(* Logix 5000 AddOnInstructionDefinition export Banner_K50ProTouch_Param_v4; software revision 33.00; part 2 of 2 *)
(* tags used below, declared in another part *)
   K50ProTouch : Banner_K50ProTouch_v4;
   Port_Data : Banner_IOL_Port_v4;
   Port : DINT;
   Local_Control : DINT;
   Command_Being_Processed : BOOL;
   Update_Archive : BOOL;
   Index_Write_Inprocess : INT;
   Inprocess_Index : DINT;
   SP_Index : DINT;   // State Parameters Index
   SP_W_Index : DINT;
(* Banner_K50ProTouch_Param_v4, continued *)

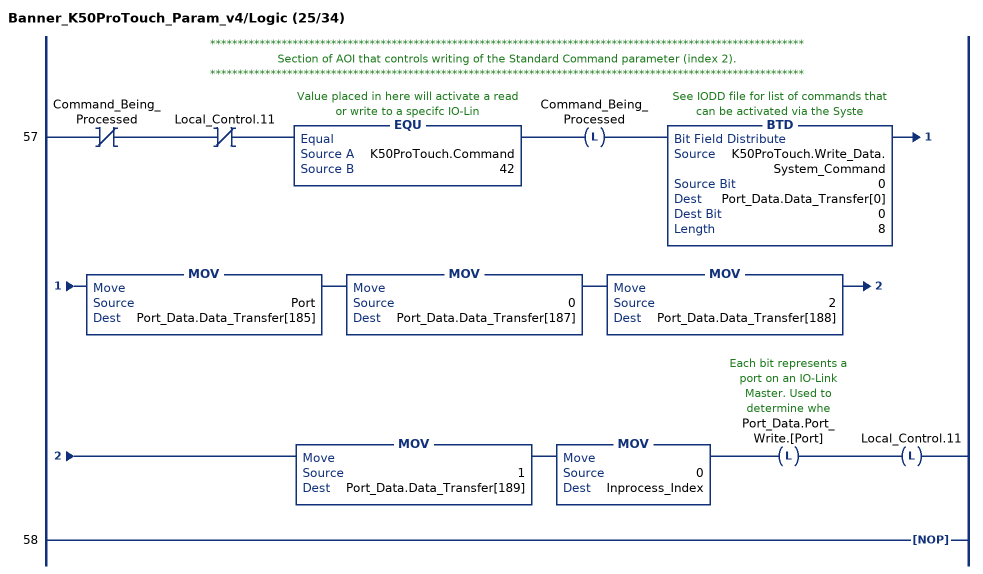
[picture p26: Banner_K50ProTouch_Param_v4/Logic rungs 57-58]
   // ************************************************************************************************************
   // Section of AOI that controls writing of the Standard Command parameter (index 2).
   // ************************************************************************************************************
   57: XIO(Command_Being_Processed)XIO(Local_Control.11)EQU(K50ProTouch.Command,42)OTL(Command_Being_Processed)BTD(K50ProTouch.Write_Data.System_Command,0,Port_Data.Data_Transfer[0],0,8)MOV(Port,Port_Data.Data_Transfer[185])MOV(0,Port_Data.Data_Transfer[187])MOV(2,Port_Data.Data_Transfer[188])MOV(1,Port_Data.Data_Transfer[189])MOV(0,Inprocess_Index)OTL(Port_Data.Port_Write.[Port])OTL(Local_Control.11);
   58: NOP();
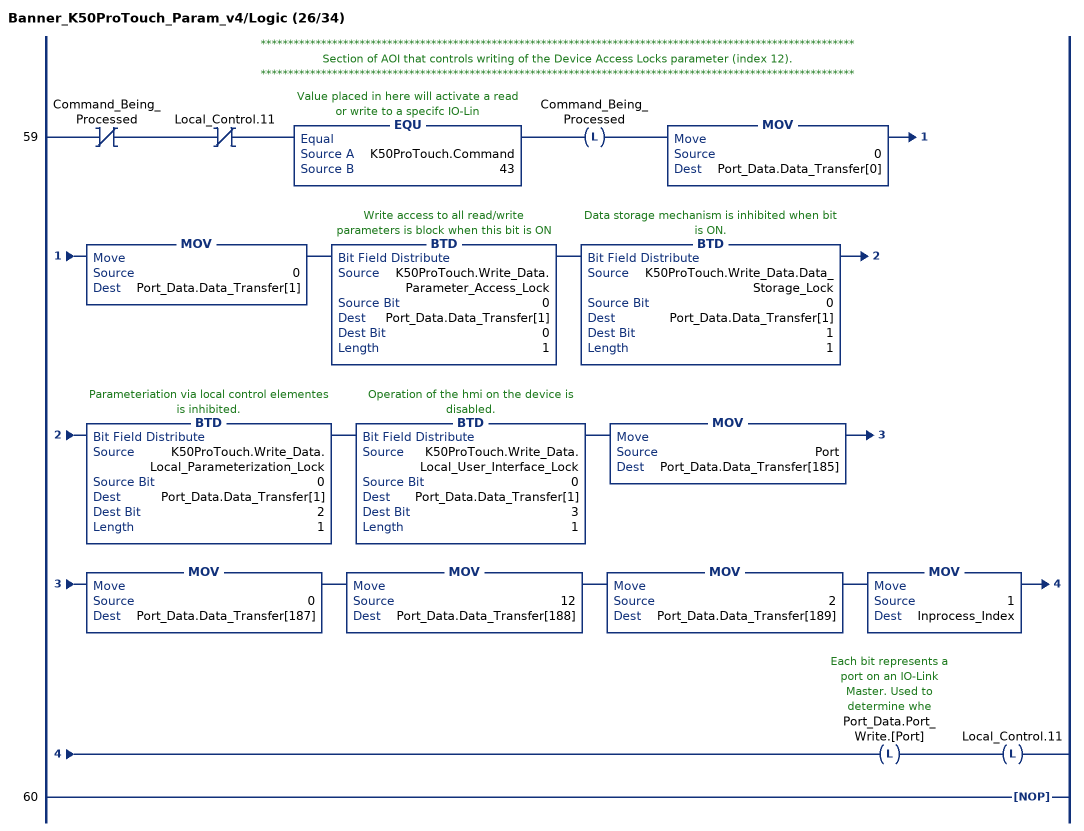
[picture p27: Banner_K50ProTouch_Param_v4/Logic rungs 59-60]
   // ************************************************************************************************************
   // Section of AOI that controls writing of the Device Access Locks parameter (index 12).
   // ************************************************************************************************************
   59: XIO(Command_Being_Processed)XIO(Local_Control.11)EQU(K50ProTouch.Command,43)OTL(Command_Being_Processed)MOV(0,Port_Data.Data_Transfer[0])MOV(0,Port_Data.Data_Transfer[1])BTD(K50ProTouch.Write_Data.Parameter_Access_Lock,0,Port_Data.Data_Transfer[1],0,1)BTD(K50ProTouch.Write_Data.Data_Storage_Lock,0,Port_Data.Data_Transfer[1],1,1)BTD(K50ProTouch.Write_Data.Local_Parameterization_Lock,0,Port_Data.Data_Transfer[1],2,1)BTD(K50ProTouch.Write_Data.Local_User_Interface_Lock,0,Port_Data.Data_Transfer[1],3,1)MOV(Port,Port_Data.Data_Transfer[185])MOV(0,Port_Data.Data_Transfer[187])MOV(12,Port_Data.Data_Transfer[188])MOV(2,Port_Data.Data_Transfer[189])MOV(1,Inprocess_Index)OTL(Port_Data.Port_Write.[Port])OTL(Local_Control.11);
   60: NOP();
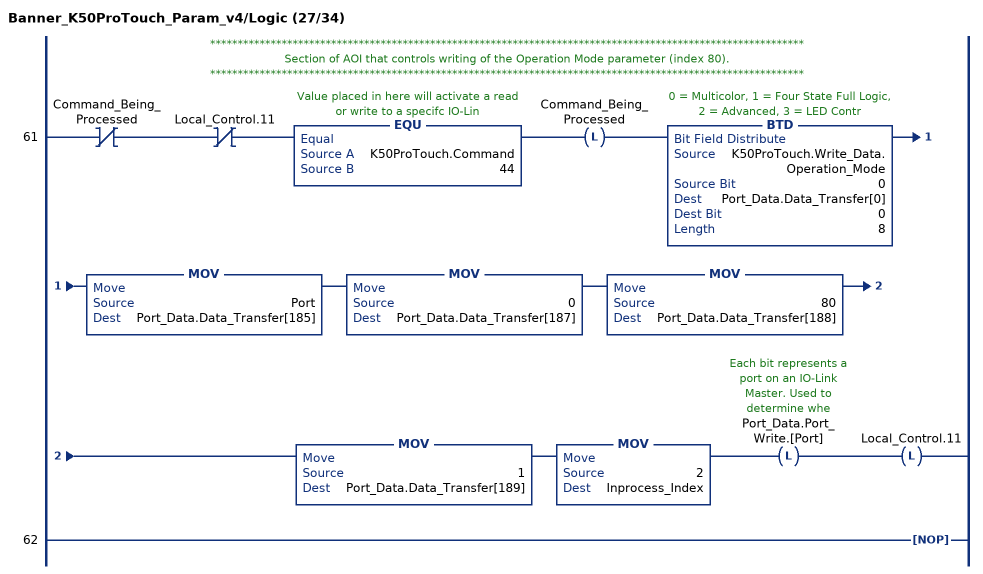
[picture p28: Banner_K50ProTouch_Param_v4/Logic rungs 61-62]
   // ************************************************************************************************************
   // Section of AOI that controls writing of the Operation Mode parameter (index 80).
   // ************************************************************************************************************
   61: XIO(Command_Being_Processed)XIO(Local_Control.11)EQU(K50ProTouch.Command,44)OTL(Command_Being_Processed)BTD(K50ProTouch.Write_Data.Operation_Mode,0,Port_Data.Data_Transfer[0],0,8)MOV(Port,Port_Data.Data_Transfer[185])MOV(0,Port_Data.Data_Transfer[187])MOV(80,Port_Data.Data_Transfer[188])MOV(1,Port_Data.Data_Transfer[189])MOV(2,Inprocess_Index)OTL(Port_Data.Port_Write.[Port])OTL(Local_Control.11);
   62: NOP();
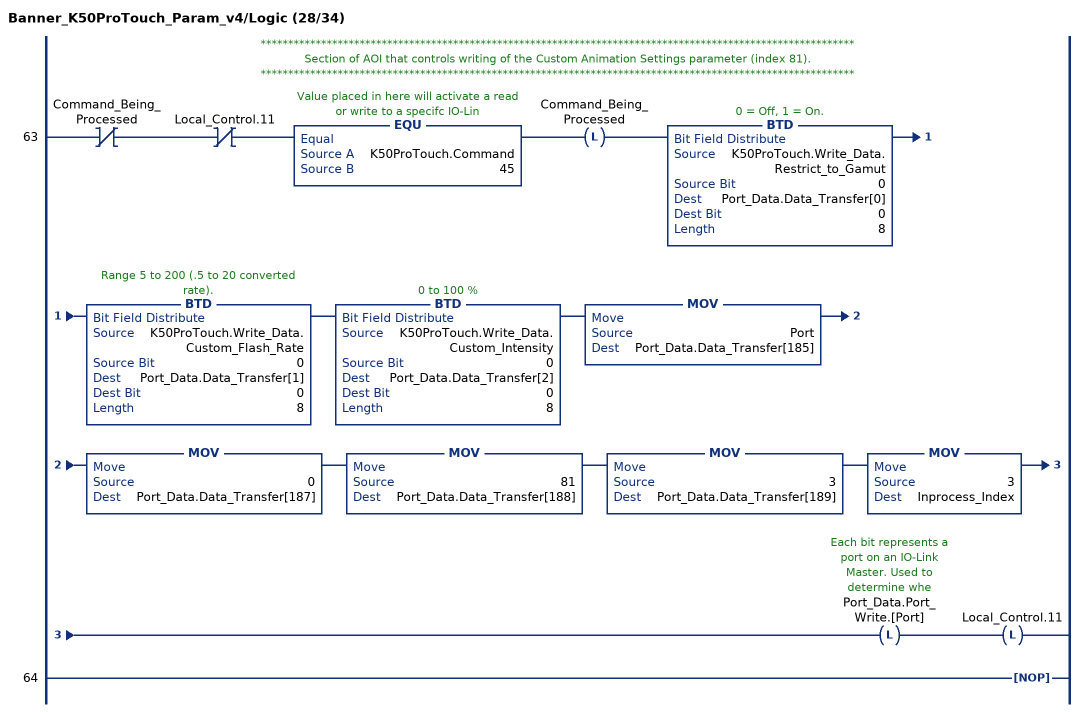
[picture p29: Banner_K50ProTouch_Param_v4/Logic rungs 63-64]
   // ************************************************************************************************************
   // Section of AOI that controls writing of the Custom Animation Settings parameter (index 81).
   // ************************************************************************************************************
   63: XIO(Command_Being_Processed)XIO(Local_Control.11)EQU(K50ProTouch.Command,45)OTL(Command_Being_Processed)BTD(K50ProTouch.Write_Data.Restrict_to_Gamut,0,Port_Data.Data_Transfer[0],0,8)BTD(K50ProTouch.Write_Data.Custom_Flash_Rate,0,Port_Data.Data_Transfer[1],0,8)BTD(K50ProTouch.Write_Data.Custom_Intensity,0,Port_Data.Data_Transfer[2],0,8)MOV(Port,Port_Data.Data_Transfer[185])MOV(0,Port_Data.Data_Transfer[187])MOV(81,Port_Data.Data_Transfer[188])MOV(3,Port_Data.Data_Transfer[189])MOV(3,Inprocess_Index)OTL(Port_Data.Port_Write.[Port])OTL(Local_Control.11);
   64: NOP();
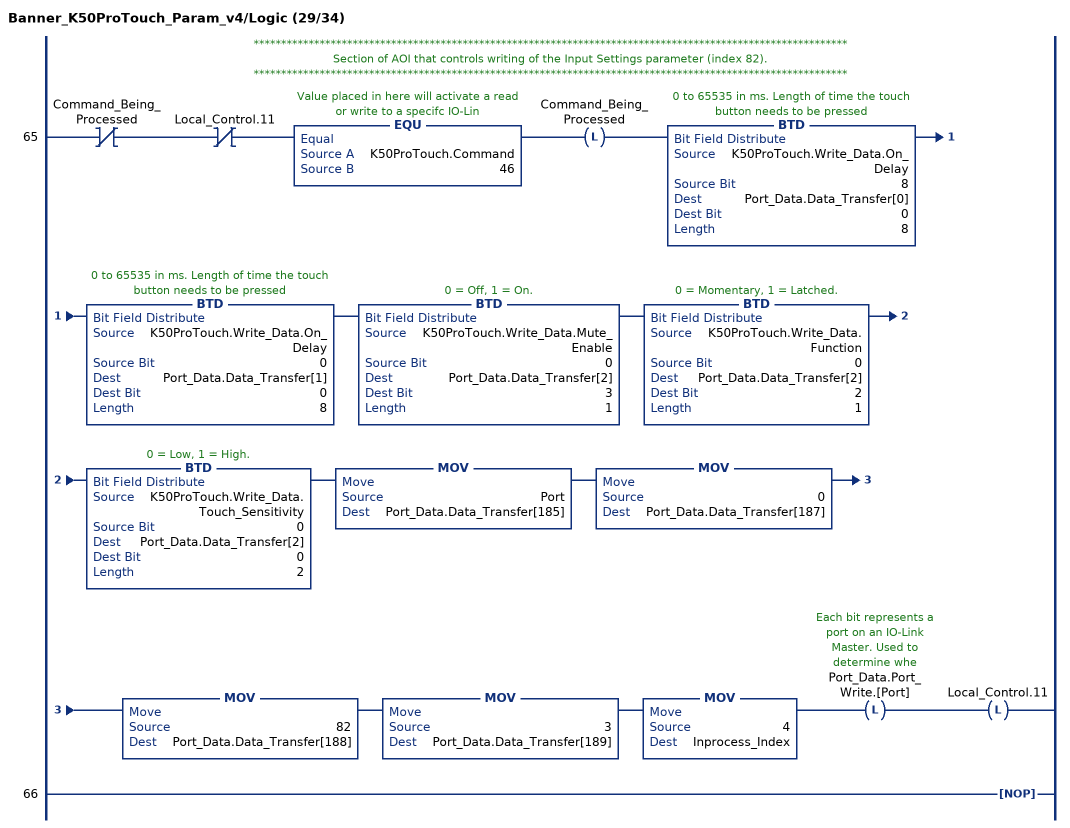
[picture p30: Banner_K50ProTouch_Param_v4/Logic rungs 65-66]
   // ************************************************************************************************************
   // Section of AOI that controls writing of the Input Settings parameter (index 82).
   // ************************************************************************************************************
   65: XIO(Command_Being_Processed)XIO(Local_Control.11)EQU(K50ProTouch.Command,46)OTL(Command_Being_Processed)BTD(K50ProTouch.Write_Data.On_Delay,8,Port_Data.Data_Transfer[0],0,8)BTD(K50ProTouch.Write_Data.On_Delay,0,Port_Data.Data_Transfer[1],0,8)BTD(K50ProTouch.Write_Data.Mute_Enable,0,Port_Data.Data_Transfer[2],3,1)BTD(K50ProTouch.Write_Data.Function,0,Port_Data.Data_Transfer[2],2,1)BTD(K50ProTouch.Write_Data.Touch_Sensitivity,0,Port_Data.Data_Transfer[2],0,2)MOV(Port,Port_Data.Data_Transfer[185])MOV(0,Port_Data.Data_Transfer[187])MOV(82,Port_Data.Data_Transfer[188])MOV(3,Port_Data.Data_Transfer[189])MOV(4,Inprocess_Index)OTL(Port_Data.Port_Write.[Port])OTL(Local_Control.11);
   66: NOP();
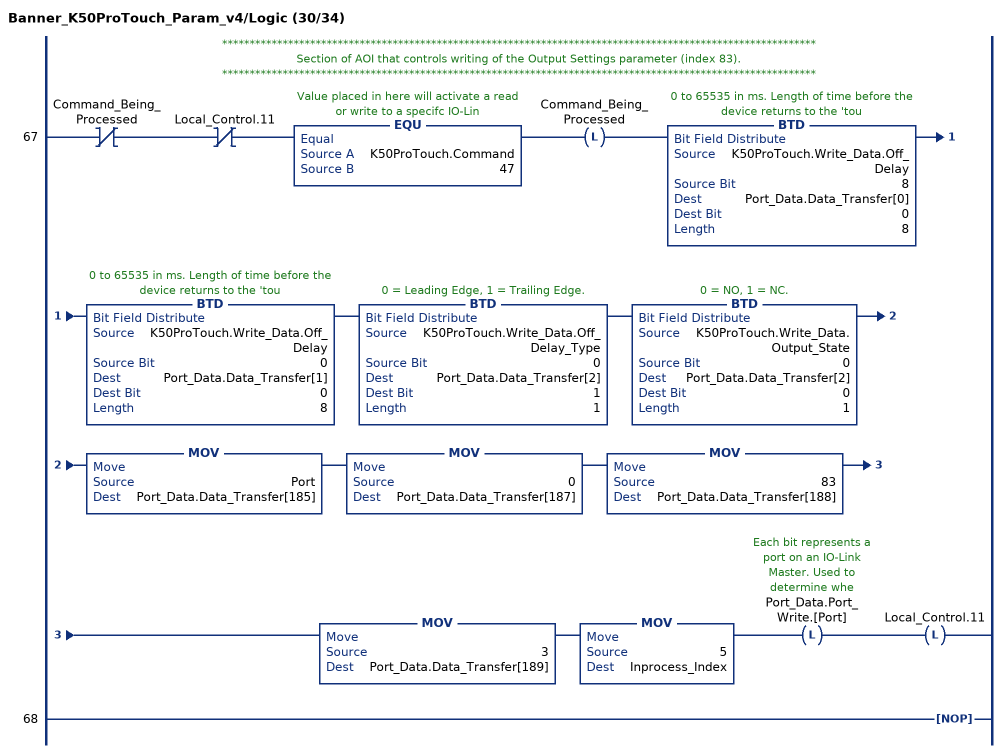
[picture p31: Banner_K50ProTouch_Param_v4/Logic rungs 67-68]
   // ************************************************************************************************************
   // Section of AOI that controls writing of the Output Settings parameter (index 83).
   // ************************************************************************************************************
   67: XIO(Command_Being_Processed)XIO(Local_Control.11)EQU(K50ProTouch.Command,47)OTL(Command_Being_Processed)BTD(K50ProTouch.Write_Data.Off_Delay,8,Port_Data.Data_Transfer[0],0,8)BTD(K50ProTouch.Write_Data.Off_Delay,0,Port_Data.Data_Transfer[1],0,8)BTD(K50ProTouch.Write_Data.Off_Delay_Type,0,Port_Data.Data_Transfer[2],1,1)BTD(K50ProTouch.Write_Data.Output_State,0,Port_Data.Data_Transfer[2],0,1)MOV(Port,Port_Data.Data_Transfer[185])MOV(0,Port_Data.Data_Transfer[187])MOV(83,Port_Data.Data_Transfer[188])MOV(3,Port_Data.Data_Transfer[189])MOV(5,Inprocess_Index)OTL(Port_Data.Port_Write.[Port])OTL(Local_Control.11);
   68: NOP();
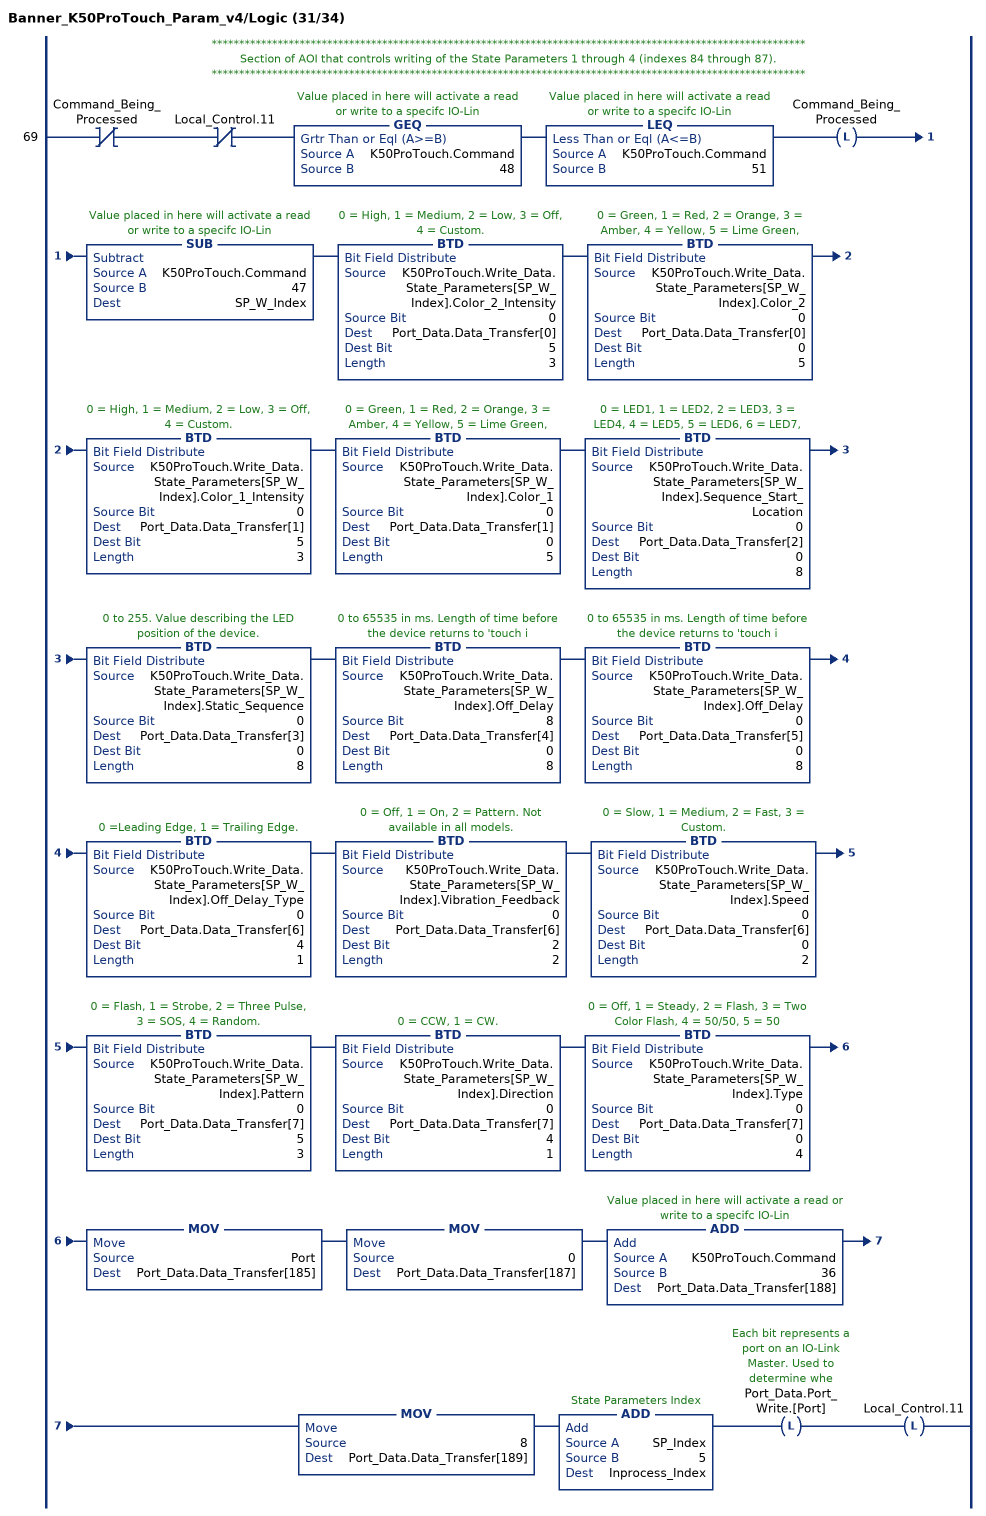
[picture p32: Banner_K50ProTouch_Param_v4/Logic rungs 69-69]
   // ************************************************************************************************************
   // Section of AOI that controls writing of the State Parameters 1 through 4 (indexes 84 through 87).
   // ************************************************************************************************************
   69: XIO(Command_Being_Processed)XIO(Local_Control.11)GEQ(K50ProTouch.Command,48)LEQ(K50ProTouch.Command,51)OTL(Command_Being_Processed)SUB(K50ProTouch.Command,47,SP_W_Index)BTD(K50ProTouch.Write_Data.State_Parameters[SP_W_Index].Color_2_Intensity,0,Port_Data.Data_Transfer[0],5,3)BTD(K50ProTouch.Write_Data.State_Parameters[SP_W_Index].Color_2,0,Port_Data.Data_Transfer[0],0,5)BTD(K50ProTouch.Write_Data.State_Parameters[SP_W_Index].Color_1_Intensity,0,Port_Data.Data_Transfer[1],5,3)BTD(K50ProTouch.Write_Data.State_Parameters[SP_W_Index].Color_1,0,Port_Data.Data_Transfer[1],0,5)BTD(K50ProTouch.Write_Data.State_Parameters[SP_W_Index].Sequence_Start_Location,0,Port_Data.Data_Transfer[2],0,8)BTD(K50ProTouch.Write_Data.State_Parameters[SP_W_Index].Static_Sequence,0,Port_Data.Data_Transfer[3],0,8)BTD(K50ProTouch.Write_Data.State_Parameters[SP_W_Index].Off_Delay,8,Port_Data.Data_Transfer[4],0,8)BTD(K50ProTouch.Write_Data.State_Parameters[SP_W_Index].Off_Delay,0,Port_Data.Data_Transfer[5],0,8)BTD(K50ProTouch.Write_Data.State_Parameters[SP_W_Index].Off_Delay_Type,0,Port_Data.Data_Transfer[6],4,1)BTD(K50ProTouch.Write_Data.State_Parameters[SP_W_Index].Vibration_Feedback,0,Port_Data.Data_Transfer[6],2,2)BTD(K50ProTouch.Write_Data.State_Parameters[SP_W_Index].Speed,0,Port_Data.Data_Transfer[6],0,2)BTD(K50ProTouch.Write_Data.State_Parameters[SP_W_Index].Pattern,0,Port_Data.Data_Transfer[7],5,3)BTD(K50ProTouch.Write_Data.State_Parameters[SP_W_Index].Direction,0,Port_Data.Data_Transfer[7],4,1)BTD(K50ProTouch.Write_Data.State_Parameters[SP_W_Index].Type,0,Port_Data.Data_Transfer[7],0,4)MOV(Port,Port_Data.Data_Transfer[185])MOV(0,Port_Data.Data_Transfer[187])ADD(K50ProTouch.Command,36,Port_Data.Data_Transfer[188])MOV(8,Port_Data.Data_Transfer[189])ADD(SP_Index,5,Inprocess_Index)OTL(Port_Data.Port_Write.[Port])OTL(Local_Control.11);
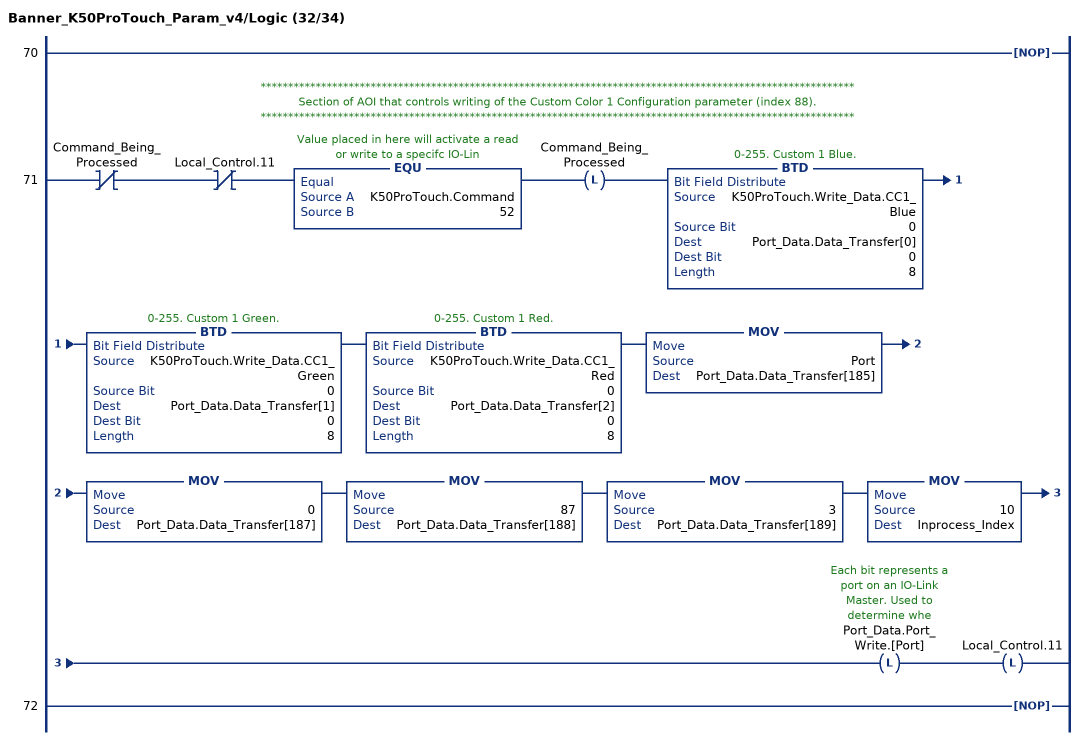
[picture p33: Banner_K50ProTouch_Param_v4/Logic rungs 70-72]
   70: NOP();
   // ************************************************************************************************************
   // Section of AOI that controls writing of the Custom Color 1 Configuration parameter (index 88).
   // ************************************************************************************************************
   71: XIO(Command_Being_Processed)XIO(Local_Control.11)EQU(K50ProTouch.Command,52)OTL(Command_Being_Processed)BTD(K50ProTouch.Write_Data.CC1_Blue,0,Port_Data.Data_Transfer[0],0,8)BTD(K50ProTouch.Write_Data.CC1_Green,0,Port_Data.Data_Transfer[1],0,8)BTD(K50ProTouch.Write_Data.CC1_Red,0,Port_Data.Data_Transfer[2],0,8)MOV(Port,Port_Data.Data_Transfer[185])MOV(0,Port_Data.Data_Transfer[187])MOV(87,Port_Data.Data_Transfer[188])MOV(3,Port_Data.Data_Transfer[189])MOV(10,Inprocess_Index)OTL(Port_Data.Port_Write.[Port])OTL(Local_Control.11);
   72: NOP();
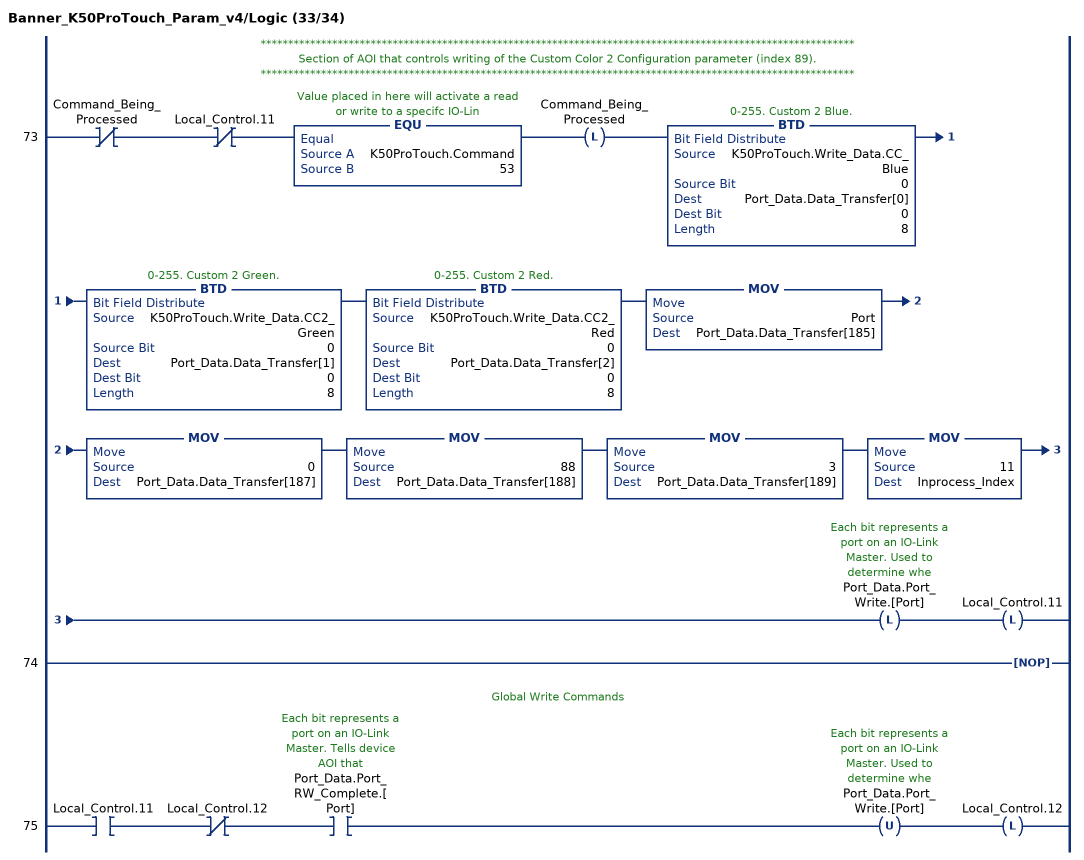
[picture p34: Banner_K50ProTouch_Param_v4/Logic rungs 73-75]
   // ************************************************************************************************************
   // Section of AOI that controls writing of the Custom Color 2 Configuration parameter (index 89).
   // ************************************************************************************************************
   73: XIO(Command_Being_Processed)XIO(Local_Control.11)EQU(K50ProTouch.Command,53)OTL(Command_Being_Processed)BTD(K50ProTouch.Write_Data.CC_Blue,0,Port_Data.Data_Transfer[0],0,8)BTD(K50ProTouch.Write_Data.CC2_Green,0,Port_Data.Data_Transfer[1],0,8)BTD(K50ProTouch.Write_Data.CC2_Red,0,Port_Data.Data_Transfer[2],0,8)MOV(Port,Port_Data.Data_Transfer[185])MOV(0,Port_Data.Data_Transfer[187])MOV(88,Port_Data.Data_Transfer[188])MOV(3,Port_Data.Data_Transfer[189])MOV(11,Inprocess_Index)OTL(Port_Data.Port_Write.[Port])OTL(Local_Control.11);
   74: NOP();
   // Global Write Commands
   75: XIC(Local_Control.11)XIO(Local_Control.12)XIC(Port_Data.Port_RW_Complete.[Port])OTU(Port_Data.Port_Write.[Port])OTL(Local_Control.12);
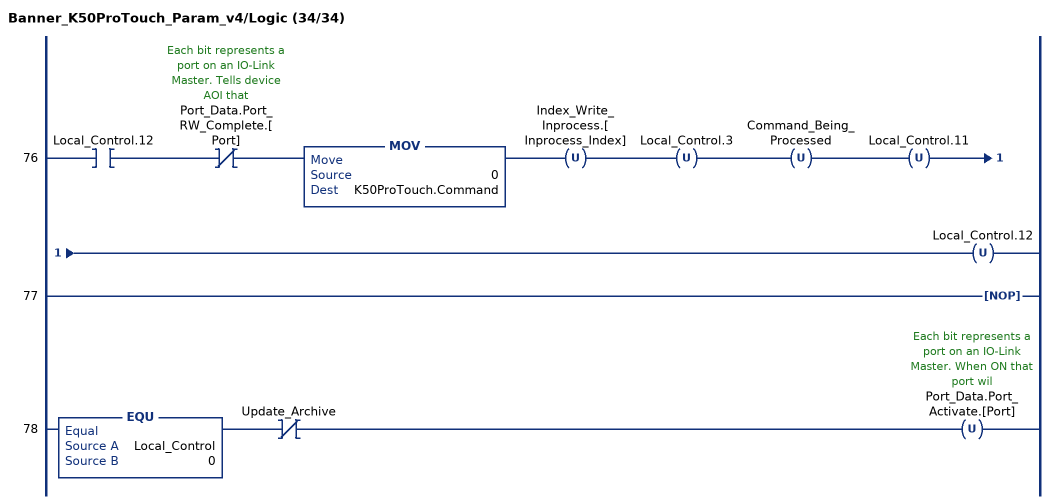
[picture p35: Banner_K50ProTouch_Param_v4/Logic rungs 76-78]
   76: XIC(Local_Control.12)XIO(Port_Data.Port_RW_Complete.[Port])MOV(0,K50ProTouch.Command)OTU(Index_Write_Inprocess.[Inprocess_Index])OTU(Local_Control.3)OTU(Command_Being_Processed)OTU(Local_Control.11)OTU(Local_Control.12);
   77: NOP();
   78: EQU(Local_Control,0)XIO(Update_Archive)OTU(Port_Data.Port_Activate.[Port]);
END_ROUTINE
END_ADD_ON_INSTRUCTION
